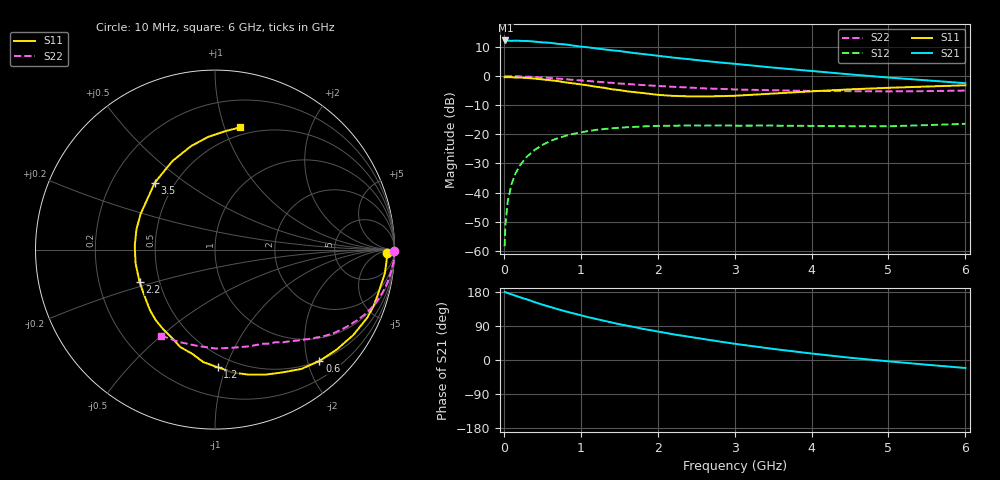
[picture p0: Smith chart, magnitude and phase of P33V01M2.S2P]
! SIEMENS Small Signal Semiconductors
! BFP181
! Si NPN RF Bipolar Junction Transistor in SOT143
! VCE = 3 V  IC = 1.2 mA
! Common Emitter S-Parameters:  March  1996
# GHz  S  MA  R  50
!  f  S11  S21  S12  S22
! GHz  MAG  ANG  MAG  ANG  MAG  ANG  MAG  ANG
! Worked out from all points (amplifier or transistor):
!   36 points, 10 MHz to 6 GHz, reference 50 ohm
!   highest |S21| = 12.2 dB at 20 MHz (marker M1)
!   |S21| within 3 dB of that: start of sweep to 1.285 GHz
!   unconditionally stable (mu >= 1): 2.909 GHz to end of sweep
!   at 250 MHz: K = 0.09, MSG = 20.7 dB, |S12| = -29.3 dB
!   at 1.4 GHz: K = 0.53, MSG = 13.4 dB, |S12| = -17.9 dB
!   at 6 GHz: K = 1.24, MAG = 4.0 dB, |S12| = -16.4 dB
!   S11 on the Smith chart (normalised r, x): 10 MHz: 39, -16; 600 MHz: 0.49, -2.21; 1.2 GHz: 0.41, -0.94; 2.2 GHz: 0.39, -0.18; 3.5 GHz: 0.39, +0.39; 6 GHz: 0.43, +1.13
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0.01  0.9572 -1.0  4.061 179.5  0.0012 88.4  0.9979 -0.3
0.02  0.9582 -1.8  4.095 179.2  0.0027 94.0  0.9902 -0.7
0.05  0.958 -3.9  4.085 176.6  0.007 91.1  0.9964 -1.8
0.1  0.9556 -8.0  4.026 173.3  0.0139 84.2  0.9982 -3.7
0.15  0.9452 -12.2  4.071 169.7  0.0211 81.4  0.9926 -5.6
0.2  0.9409 -15.9  4.045 166.2  0.0282 80.2  0.9882 -7.4
0.3  0.9293 -24.1  4.011 160.0  0.0413 74.9  0.9775 -11.0
0.4  0.9057 -31.7  3.916 152.8  0.0538 69.3  0.9638 -14.4
0.6  0.8508 -46.9  3.736 140.1  0.0767 60.3  0.9282 -20.8
0.8  0.7807 -61.2  3.5 128.4  0.0941 52.0  0.8848 -26.4
1.1  0.6909 -82.1  3.119 112.8  0.114 41.3  0.822 -33.5
1.2  0.6559 -88.6  2.989 108.3  0.1193 37.9  0.8044 -35.7
1.4  0.5948 -102.2  2.779 99.1  0.1271 32.6  0.766 -39.4
1.6  0.5479 -115.8  2.587 90.6  0.1324 28.1  0.7338 -42.5
1.8  0.5134 -130.1  2.401 82.5  0.1367 24.3  0.7033 -45.5
2.2  0.4576 -156.7  2.08 68.0  0.1405 17.4  0.6548 -51.4
2.8  0.4519 165.8  1.719 48.9  0.1423 10.4  0.6058 -59.8
3.5  0.5015 132.0  1.4 29.3  0.1412 5.6  0.5718 -70.4
4  0.5474 115.7  1.225 17.1  0.1394 3.6  0.5559 -79.5
4.5  0.5924 102.9  1.07 6.0  0.1381 2.0  0.5511 -89.7
5.5  0.6622 85.1  0.845 -12.5  0.1439 4.3  0.5519 -110.9
6  0.6957 78.3  0.755 -21.1  0.1516 4.1  0.565 -121.9
